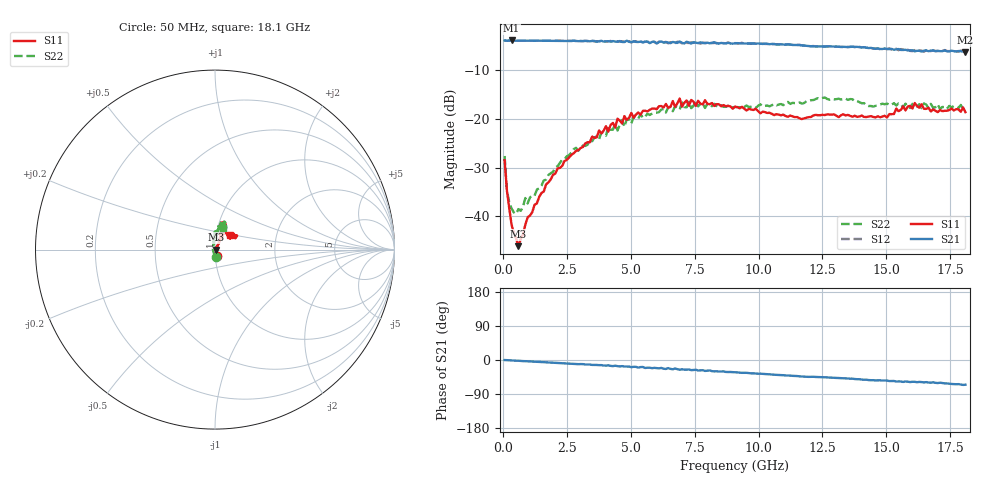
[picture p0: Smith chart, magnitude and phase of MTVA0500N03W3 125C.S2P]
! Network Analyzer HP8720D.06.14 Serial No. US36140669
!  8 Jul 2005  08:33:24
! Frequency  S11  S21  S12  S22
# HZ  S  DB R 50
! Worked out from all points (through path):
!   201 points, 50 MHz to 18.1 GHz, reference 50 ohm
!   highest |S21| = -3.82 dB at 320.8 MHz (marker M1); lowest = -6.2 dB at 18.1 GHz (marker M2)
!   group delay of S21, straight-line fit = 10.1 ps
!   lowest |S11| = -46.2 dB at 591.5 MHz (marker M3), VSWR 1.01, Z = 50.5 + j0.0347 ohm
!   |S11| at or under -10 dB: start of sweep to end of sweep
!   |S22| runs from -39.5 to -15.6 dB; largest |S21 - S12| = 0.027
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5e7  -28.43 -74.6  -3.82 -0.1  -3.82 0.1  -27.59 -80.5
1.4025e8  -34.71 -66.0  -3.89 -0.4  -3.86 -0.5  -34.66 -115.0
3.2075e8  -41.68 -48.4  -3.82 -1.0  -3.84 -1.1  -38.40 -149.0
5.915e8  -46.15 4.0  -3.85 -2.0  -3.87 -2.0  -38.52 173.1
8.6225e8  -41.73 36.7  -3.87 -3.0  -3.87 -3.1  -36.24 156.3
9.525e8  -40.20 43.6  -3.88 -3.3  -3.86 -3.4  -37.36 145.0
1.6745e9  -33.44 54.9  -3.88 -6.0  -3.88 -6.1  -32.45 115.8
3.1185e9  -25.74 63.6  -3.94 -10.9  -3.97 -11.3  -25.44 99.4
4.021e9  -21.47 65.9  -3.99 -14.9  -4.02 -14.1  -23.42 90.3
4.11125e9  -22.59 65.6  -3.97 -14.1  -4.01 -15.2  -21.58 89.7
4.47225e9  -19.91 62.4  -4.09 -16.2  -3.97 -15.4  -22.35 93.0
4.65275e9  -20.92 62.7  -4.13 -16.2  -3.98 -17.1  -20.18 91.7
4.743e9  -19.39 66.6  -4.15 -17.2  -4.10 -16.5  -21.59 87.7
6.09675e9  -17.35 68.0  -4.15 -22.0  -4.05 -21.9  -18.57 80.2
6.909e9  -15.77 72.3  -4.04 -25.7  -4.16 -24.2  -18.05 74.5
6.99925e9  -17.45 71.9  -4.31 -24.4  -4.41 -26.1  -16.54 75.6
7.54075e9  -17.30 70.3  -4.27 -25.6  -4.13 -27.9  -16.27 78.3
9.075e9  -17.43 75.6  -4.38 -32.4  -4.36 -32.4  -17.51 70.3
1.21435e10  -19.25 60.4  -5.01 -44.3  -4.96 -44.4  -16.08 71.7
1.512175e10  -18.97 39.1  -5.60 -55.6  -5.44 -55.2  -17.08 72.9
1.61145e10  -16.69 32.4  -6.06 -57.6  -5.80 -57.9  -17.73 70.9
1.81e10  -18.58 44.4  -6.22 -65.1  -6.37 -65.9  -17.92 70.6
